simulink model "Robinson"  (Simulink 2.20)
settings: Solver=ode3  StartTime=0.0  StopTime=1  FixedStep=0.001  MaxStep=0.001  RelTol=1e-3  AbsTol=1e-6

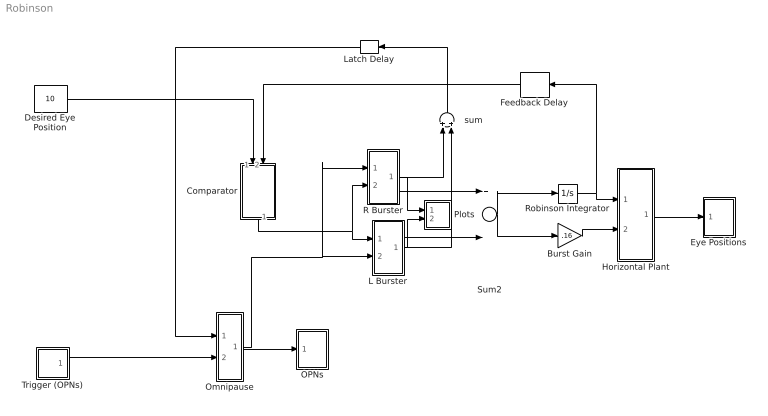
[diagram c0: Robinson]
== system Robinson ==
  Burst Gain : Gain  Gain=.16
  Comparator : Subsystem  Orientation=down
  Desired Eye Position : Constant  Value=10
  Eye Positions : Subsystem  mask(Graph scope.){}
      mask help: Graph scope using MATLAB graph window. Enter plotting ranges and line type.
      mask init:
      | color = @4; ax = [0, @1, @2, @3]; dt = -1;
  Feedback Delay : TransportDelay  Orientation=left  DelayTime=.002  InitialInput=0  BufferSize=1024
  Horizontal Plant : Subsystem
  L Burster : Subsystem
  Latch Delay : TransportDelay  Orientation=left  DelayTime=.002  InitialInput=00  BufferSize=1024
  OPNs : Subsystem  mask(Graph scope.){}
      mask help: Graph scope using MATLAB graph window. Enter plotting ranges and line type.
      mask init:
      | color = @4; ax = [0, @1, @2, @3]; dt = -1;
  Omnipause : Subsystem
  Plots : Subsystem
  R Burster : Subsystem
  Robinson Integrator : Integrator  ExternalReset=none  InitialConditionSource=internal  InitialCondition=0  LimitOutput=off  UpperSaturationLimit=inf  LowerSaturationLimit=-inf  ShowSaturationPort=off  ShowStatePort=off  AbsoluteTolerance=auto
  Sum2 : Sum  Inputs=+-
  Trigger (OPNs) : Subsystem  mask(Pulse Generator){period=1, duty=3, amplitude=1, start=.1}
      mask prompts: period "Period (secs):"; duty "Duty cycle (% of period):"; start "Start time:"
      mask help: Pulse Generator
  sum : Sum  Orientation=up  Inputs=++
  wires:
  Trigger (OPNs)/1(out1) -> Omnipause/2(in_2)
  Desired Eye Position/1 -> Comparator/1(in_1)
  L Burster/1(out_1) -> sum/2, Sum2/2, Plots/2(in_2)
  R Burster/1(out_2) -> Sum2/1, Plots/1(in_1), sum/1
  Omnipause/1(out_1) -> OPNs/1(x), R Burster/1(in_2), L Burster/2(in_2)
  Feedback Delay/1 -> Comparator/2(in_2)
  Robinson Integrator/1 -> Feedback Delay/1, Horizontal Plant/1(in_1)
  Latch Delay/1 -> Omnipause/1(in_1)
  sum/1 -> Latch Delay/1
  Comparator/1(out_1) -> R Burster/2(in_1), L Burster/1(in_1)
  Horizontal Plant/1(out_1) -> Eye Positions/1(x)
  Sum2/1 -> Burst Gain/1, Robinson Integrator/1
  Burst Gain/1 -> Horizontal Plant/2(in_2)

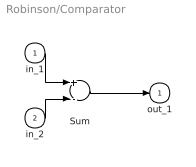
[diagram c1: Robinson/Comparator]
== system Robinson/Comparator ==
  in_1 : Inport  Port=1  PortWidth=-1  SampleTime=-1
  in_2 : Inport  Port=2  PortWidth=-1  SampleTime=-1
  Sum : Sum  Inputs=+-
  out_1 : Outport  Port=1  InitialOutput=0
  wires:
  in_2/1 -> Sum/2
  in_1/1 -> Sum/1
  Sum/1 -> out_1/1

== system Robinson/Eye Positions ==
  x : Inport  Port=1  PortWidth=-1  SampleTime=-1
  "S-function M-file which plots lines " : S-Function  FunctionName=sfuny  Parameters=ax, color,dt  PortCounts=[]  SFunctionModules=''
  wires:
  x/1 -> "S-function M-file which plots lines "/1

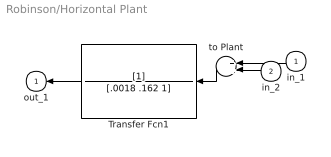
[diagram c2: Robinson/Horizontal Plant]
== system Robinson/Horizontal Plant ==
  in_1 : Inport  Orientation=left  Port=1  PortWidth=-1  SampleTime=-1
  in_2 : Inport  Orientation=left  Port=2  PortWidth=-1  SampleTime=-1
  Transfer Fcn1 : TransferFcn  Orientation=left  Numerator=[1]  Denominator=[.0018 .162 1]
  to Plant : Sum  Orientation=left  Inputs=++
  out_1 : Outport  Orientation=left  Port=1  InitialOutput=0
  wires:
  Transfer Fcn1/1 -> out_1/1
  in_2/1 -> to Plant/2
  in_1/1 -> to Plant/1
  to Plant/1 -> Transfer Fcn1/1

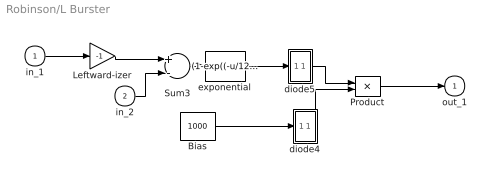
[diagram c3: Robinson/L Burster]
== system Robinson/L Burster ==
  in_1 : Inport  Port=1  PortWidth=-1  SampleTime=-1
  in_2 : Inport  Port=2  PortWidth=-1  SampleTime=-1
  Bias : Constant  Value=1000
  Leftward-izer : Gain  Gain=-1
  Product : Product  Inputs=2
  Sum3 : Sum  Inputs=+-
  diode4 : Subsystem
  diode5 : Subsystem
  exponential : Fcn  Expr=(1-exp((-u/12)))
  out_1 : Outport  Port=1  InitialOutput=0
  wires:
  Product/1 -> out_1/1
  in_2/1 -> Sum3/2
  Sum3/1 -> exponential/1
  Bias/1 -> diode4/1(in_1)
  diode5/1(out_1) -> Product/1
  exponential/1 -> diode5/1(in_1)
  diode4/1(out_1) -> Product/2
  in_1/1 -> Leftward-izer/1
  Leftward-izer/1 -> Sum3/1

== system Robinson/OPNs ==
  x : Inport  Port=1  PortWidth=-1  SampleTime=-1
  "S-function M-file which plots lines " : S-Function  FunctionName=sfuny  Parameters=ax, color,dt  PortCounts=[]  SFunctionModules=''
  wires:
  x/1 -> "S-function M-file which plots lines "/1

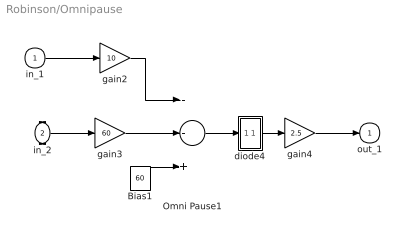
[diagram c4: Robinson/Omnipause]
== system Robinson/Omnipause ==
  in_1 : Inport  Port=1  PortWidth=-1  SampleTime=-1
  in_2 : Inport  Port=2  PortWidth=-1  SampleTime=-1
  Bias1 : Constant  Value=60
  Omni Pause1 : Sum  Inputs=--+
  diode4 : Subsystem
  gain2 : Gain  Gain=10
  gain3 : Gain  Gain=60
  gain4 : Gain  Gain=2.5
  out_1 : Outport  Port=1  InitialOutput=0
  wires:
  gain3/1 -> Omni Pause1/2
  in_2/1 -> gain3/1
  gain4/1 -> out_1/1
  diode4/1(out_1) -> gain4/1
  gain2/1 -> Omni Pause1/1
  in_1/1 -> gain2/1
  Bias1/1 -> Omni Pause1/3
  Omni Pause1/1 -> diode4/1(in_1)

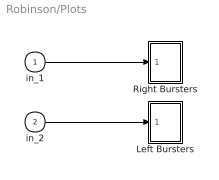
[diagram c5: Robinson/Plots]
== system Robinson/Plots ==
  in_1 : Inport  Port=1  PortWidth=-1  SampleTime=-1
  in_2 : Inport  Port=2  PortWidth=-1  SampleTime=-1
  Left Bursters : Subsystem  mask(Graph scope.){}
      mask help: Graph scope using MATLAB graph window. Enter plotting ranges and line type.
      mask init:
      | color = @4; ax = [0, @1, @2, @3]; dt = -1;
  Right Bursters : Subsystem  mask(Graph scope.){}
      mask help: Graph scope using MATLAB graph window. Enter plotting ranges and line type.
      mask init:
      | color = @4; ax = [0, @1, @2, @3]; dt = -1;
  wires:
  in_2/1 -> Left Bursters/1(x)
  in_1/1 -> Right Bursters/1(x)

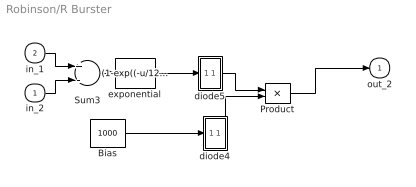
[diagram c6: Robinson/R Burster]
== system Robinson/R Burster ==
  in_2 : Inport  Port=1  PortWidth=-1  SampleTime=-1
  in_1 : Inport  Port=2  PortWidth=-1  SampleTime=-1
  Bias : Constant  Value=1000
  Product : Product  Inputs=2
  Sum3 : Sum  Inputs=+-
  diode4 : Subsystem
  diode5 : Subsystem
  exponential : Fcn  Expr=(1-exp((-u/12)))
  out_2 : Outport  Port=1  InitialOutput=0
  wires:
  Sum3/1 -> exponential/1
  Bias/1 -> diode4/1(in_1)
  in_2/1 -> Sum3/2
  in_1/1 -> Sum3/1
  diode5/1(out_1) -> Product/1
  exponential/1 -> diode5/1(in_1)
  Product/1 -> out_2/1
  diode4/1(out_1) -> Product/2

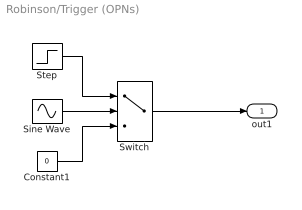
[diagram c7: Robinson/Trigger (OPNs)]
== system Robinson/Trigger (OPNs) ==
  Constant1 : Constant  Value=0
  Sine Wave : Sin  Amplitude=1  Frequency=2*pi./period  Phase=-2*pi*(start./period + duty/200 - 1/4)  SampleTime=-1
  Step : Step  Time=start  Before=0  After=amplitude
  Switch : Switch  Threshold=sin(pi*(0.5 - duty/100))
  out1 : Outport  Port=1  InitialOutput=0
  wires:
  Sine Wave/1 -> Switch/2
  Switch/1 -> out1/1
  Constant1/1 -> Switch/3
  Step/1 -> Switch/1

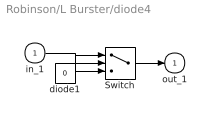
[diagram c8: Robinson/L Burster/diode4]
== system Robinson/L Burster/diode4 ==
  in_1 : Inport  Port=1  PortWidth=-1  SampleTime=-1
  Switch : Switch  Threshold=0
  diode1 : Constant  Value=0
  out_1 : Outport  Port=1  InitialOutput=0
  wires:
  in_1/1 -> Switch/2, Switch/1
  Switch/1 -> out_1/1
  diode1/1 -> Switch/3

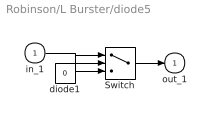
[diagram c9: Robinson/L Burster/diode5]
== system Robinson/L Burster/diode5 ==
  in_1 : Inport  Port=1  PortWidth=-1  SampleTime=-1
  Switch : Switch  Threshold=0
  diode1 : Constant  Value=0
  out_1 : Outport  Port=1  InitialOutput=0
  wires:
  diode1/1 -> Switch/3
  Switch/1 -> out_1/1
  in_1/1 -> Switch/2, Switch/1

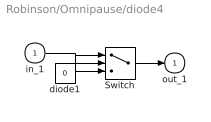
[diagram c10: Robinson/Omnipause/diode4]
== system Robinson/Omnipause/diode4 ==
  in_1 : Inport  Port=1  PortWidth=-1  SampleTime=-1
  Switch : Switch  Threshold=0
  diode1 : Constant  Value=0
  out_1 : Outport  Port=1  InitialOutput=0
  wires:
  in_1/1 -> Switch/2, Switch/1
  Switch/1 -> out_1/1
  diode1/1 -> Switch/3

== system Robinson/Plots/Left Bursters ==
  x : Inport  Port=1  PortWidth=-1  SampleTime=-1
  "S-function M-file which plots lines " : S-Function  FunctionName=sfuny  Parameters=ax, color,dt  PortCounts=[]  SFunctionModules=''
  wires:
  x/1 -> "S-function M-file which plots lines "/1

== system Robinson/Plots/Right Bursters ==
  x : Inport  Port=1  PortWidth=-1  SampleTime=-1
  "S-function M-file which plots lines " : S-Function  FunctionName=sfuny  Parameters=ax, color,dt  PortCounts=[]  SFunctionModules=''
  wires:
  x/1 -> "S-function M-file which plots lines "/1

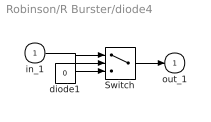
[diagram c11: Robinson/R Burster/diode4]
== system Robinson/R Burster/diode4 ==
  in_1 : Inport  Port=1  PortWidth=-1  SampleTime=-1
  Switch : Switch  Threshold=0
  diode1 : Constant  Value=0
  out_1 : Outport  Port=1  InitialOutput=0
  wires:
  in_1/1 -> Switch/2, Switch/1
  Switch/1 -> out_1/1
  diode1/1 -> Switch/3

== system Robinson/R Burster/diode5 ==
  in_1 : Inport  Port=1  PortWidth=-1  SampleTime=-1
  Switch : Switch  Threshold=0
  diode1 : Constant  Value=0
  out_1 : Outport  Port=1  InitialOutput=0
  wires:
  diode1/1 -> Switch/3
  Switch/1 -> out_1/1
  in_1/1 -> Switch/2, Switch/1
